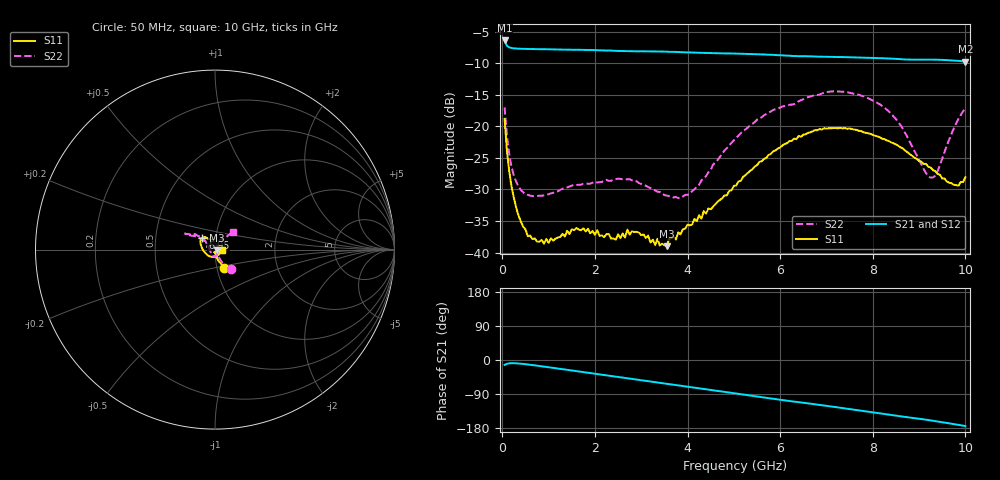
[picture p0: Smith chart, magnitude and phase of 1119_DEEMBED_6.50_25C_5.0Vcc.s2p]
!Hittite Microwave Corp.
!Digital Attenuator/PhaseShifter Rev 1.4.0
!Filename: C:\DATA\DATA\1119_DEEMBED_6.50_25C_5.0Vcc.s2p
!VNA ID: Agilent Technologies,N5224A,MY51441122,A.10.45.03
!Device type:
!2 Port Calibration.
!Temp(C): 25
!Lot Number:
!Serial Number:
!Operator:
!Misc:
!Attenuator:  6.500
# GHZ S DB R 50.0
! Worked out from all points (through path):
!   200 points, 50 MHz to 10 GHz, reference 50 ohm
!   highest |S21| = -6.41 dB at 50 MHz (marker M1); lowest = -9.8 dB at 10 GHz (marker M2)
!   group delay of S21, straight-line fit = 47 ps
!   lowest |S11| = -39.0 dB at 3.55 GHz (marker M3), VSWR 1.02, Z = 51.1 - j0.335 ohm
!   |S11| at or under -10 dB: start of sweep to end of sweep
!   |S22| runs from -31.4 to -14.5 dB; largest |S21 - S12| = 0.001
!   S11 on the Smith chart (normalised r, x): 50 MHz: 1.09, -0.22; 6.95 GHz: 0.86, +0.12; 10 GHz: 1.08, -0.00
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0.05  -18.84 -62.6  -6.41 -12.8  -6.41 -12.8  -17.01 -51.5
0.1  -23.92 -73.6  -7.25 -10.1  -7.25 -10.1  -21.51 -61.0
0.2  -29.57 -79.9  -7.60 -8.4  -7.60 -8.4  -26.42 -62.4
0.35  -34.12 -81.0  -7.71 -9.2  -7.71 -9.2  -29.52 -58.2
0.55  -37.41 -84.6  -7.76 -11.8  -7.75 -11.8  -30.86 -56.5
0.9  -38.58 -90.4  -7.80 -17.4  -7.80 -17.4  -30.93 -60.7
1.75  -36.14 -99.5  -7.90 -32.0  -7.90 -32.0  -29.09 -78.4
2.45  -37.95 -77.7  -8.06 -44.2  -8.06 -44.3  -28.34 -97.4
2.75  -37.16 -70.0  -8.11 -49.1  -8.12 -49.2  -28.38 -107.6
3.4  -38.87 -40.7  -8.16 -60.2  -8.17 -60.3  -30.39 -132.9
3.55  -38.97 -16.9  -8.18 -63.0  -8.19 -63.1  -30.97 -139.1
4.05  -35.68 10.3  -8.30 -71.5  -8.31 -71.6  -30.67 -178.2
5.05  -29.37 80.1  -8.49 -88.4  -8.51 -88.5  -21.83 137.8
5.85  -23.96 116.5  -8.69 -102.4  -8.71 -102.5  -17.40 141.9
6.7  -20.81 132.2  -8.93 -116.1  -8.94 -116.1  -15.17 149.8
6.95  -20.30 136.3  -8.98 -120.1  -8.99 -120.1  -14.67 151.7
7.7  -20.71 151.9  -9.11 -132.9  -9.12 -132.9  -15.01 152.3
8.35  -22.35 168.9  -9.27 -144.2  -9.27 -144.2  -17.67 145.5
9.15  -25.95 -135.1  -9.44 -157.5  -9.45 -157.5  -27.43 128.6
9.3  -26.95 -118.0  -9.44 -160.3  -9.46 -160.3  -28.11 101.5
9.75  -29.25 -47.4  -9.60 -169.2  -9.60 -169.2  -20.32 48.0
10  -28.06 -2.4  -9.75 -174.3  -9.76 -174.3  -17.15 45.3
